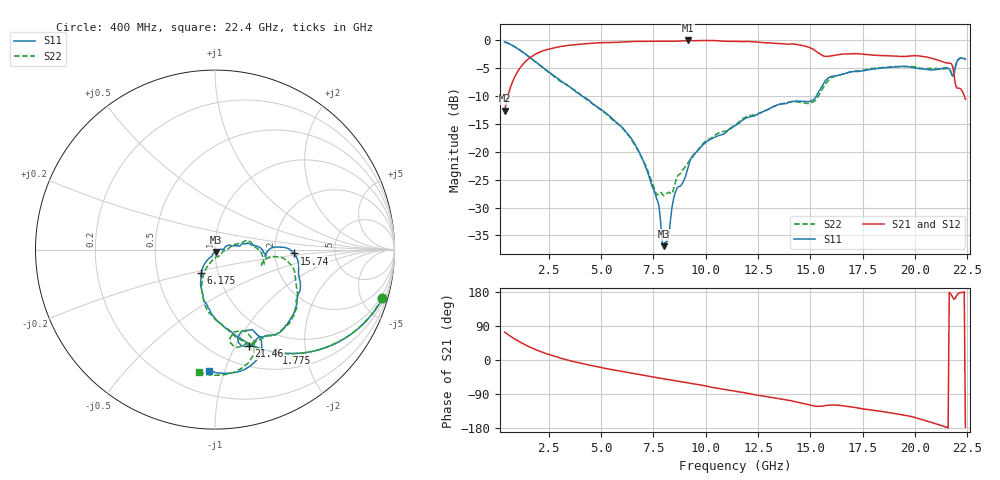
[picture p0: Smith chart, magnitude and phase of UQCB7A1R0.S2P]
!  Part Number  UQCB7A1R0	Mounting Orientation: Vertical
!  Description: RF capacitors
!  Application: Coupling, Bypass, Tuning, DC Block
!  Filters, Matching
# GHZ S DB R 50
! Freq  |S11|  S11 Ph  |S21|  S21 Ph  |S12|  S12 Ph  |S22|  S22 Ph
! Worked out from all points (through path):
!   401 points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, 400 MHz to 22.4 GHz, reference 50 ohm
!   highest |S21| = 0.00 dB at 9.145 GHz (marker M1); lowest = -12.6 dB at 400 MHz (marker M2)
!   lowest |S11| = -36.9 dB at 7.99 GHz (marker M3), VSWR 1.03, Z = 50.4 - j1.36 ohm
!   |S11| at or under -10 dB: 4.106 GHz to 15.28 GHz (11.17 GHz wide, 115 % of centre)
!   |S22| runs from -27.9 to -0.3 dB; largest |S21 - S12| = 0.0053
!   S11 on the Smith chart (normalised r, x): 400 MHz: 0.71, -6.92; 1.775 GHz: 0.73, -1.50; 6.175 GHz: 0.83, -0.23; 15.74 GHz: 2.57, -0.14; 21.46 GHz: 0.72, -1.14; 22.4 GHz: 0.36, -0.89
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0.4  -0.25 -16.3  -12.61 73.5  -12.62 73.5  -0.27 -16.2
1.06  -1.55 -39.8  -5.35 49.7  -5.37 49.6  -1.57 -39.9
1.775  -3.52 -59.2  -2.68 29.9  -2.70 29.9  -3.56 -59.6
2.765  -6.37 -77.5  -1.32 10.3  -1.33 10.3  -6.48 -78.9
4.085  -9.95 -97.4  -0.66 -9.0  -0.66 -9.0  -9.94 -99.7
6.175  -16.31 -119.9  -0.24 -31.8  -0.25 -31.8  -16.40 -114.8
7  -21.49 -126.8  -0.16 -40.2  -0.16 -40.1  -21.45 -111.0
7.77  -29.77 -114.8  -0.15 -47.5  -0.15 -47.4  -27.48 -66.7
7.99  -36.94 -72.0  -0.14 -49.4  -0.14 -49.3  -27.87 -52.7
8.21  -35.76 -21.4  -0.14 -51.5  -0.14 -51.5  -27.29 -36.8
8.54  -27.36 1.8  -0.13 -54.4  -0.12 -54.4  -25.62 -6.8
9.145  -23.03 18.2  0.00 -59.8  -0.01 -59.8  -22.06 6.5
9.915  -18.61 10.9  -0.01 -67.5  -0.01 -67.4  -18.35 14.3
11.4  -15.31 10.5  -0.16 -82.2  -0.16 -82.3  -15.26 16.1
14.095  -11.00 -6.0  -0.60 -107.5  -0.60 -107.6  -10.98 -14.7
15.085  -10.75 -3.0  -1.48 -120.2  -1.47 -120.3  -11.09 -13.9
15.745  -7.10 -2.8  -2.87 -120.0  -2.83 -120.2  -7.68 -9.6
18.77  -4.84 -43.4  -2.77 -138.9  -2.75 -139.1  -4.77 -42.2
21.465  -4.90 -70.5  -4.01 -176.9  -4.00 -177.1  -5.07 -74.8
21.795  -6.42 -72.0  -4.70 165.2  -4.69 165.0  -6.56 -76.7
22.015  -3.65 -69.1  -8.57 172.9  -8.53 172.8  -3.65 -73.4
22.4  -3.41 -92.6  -10.56 -177.7  -10.53 -177.6  -3.24 -97.4
